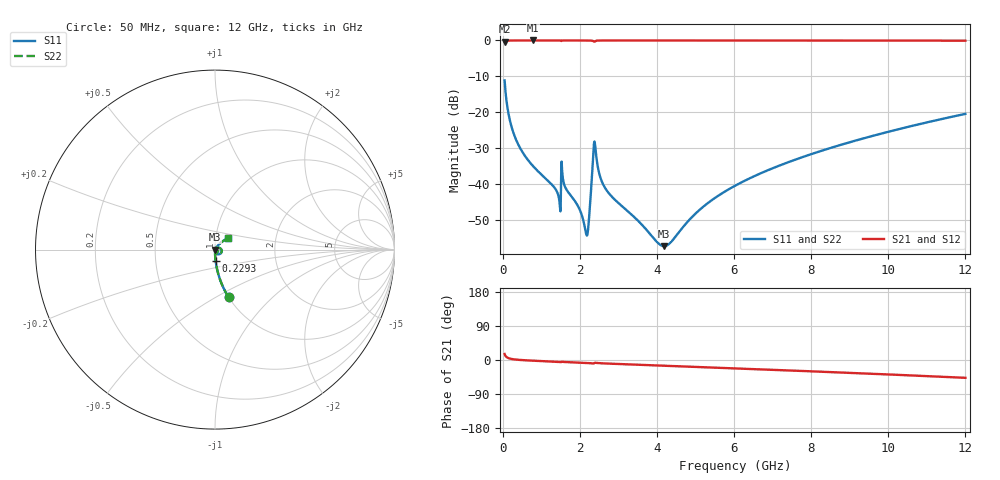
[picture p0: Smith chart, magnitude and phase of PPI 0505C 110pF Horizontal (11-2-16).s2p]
# MHz S MA R 50
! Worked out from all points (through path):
!   1601 points, 50 MHz to 12 GHz, reference 50 ohm
!   highest |S21| = -0.01 dB at 789.4 MHz (marker M1); lowest = -0.3 dB at 50 MHz (marker M2)
!   group delay of S21, straight-line fit = 11.1 ps
!   lowest |S11| = -57.4 dB at 4.188 GHz (marker M3), VSWR 1.00, Z = 50.1 - j0.0392 ohm
!   |S11| at or under -10 dB: start of sweep to end of sweep
!   |S22| runs from -57.4 to -11.1 dB; largest |S21 - S12| = 0
!   S11 on the Smith chart (normalised r, x): 50 MHz: 1.00, -0.58; 229.2 MHz: 1.00, -0.13; 12 GHz: 1.14, +0.14
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50  0.2772 -74.0  0.9606 15.9  0.9606 15.9  0.2772 -74.0
229.25  0.06265 -86.9  0.9976 2.8  0.9976 2.8  0.06265 -86.9
453.3125  0.0315 -88.9  0.9989 0.2  0.9989 0.2  0.0315 -88.9
789.4062  0.01767 -89.7  0.9991 -1.9  0.9991 -1.9  0.01767 -89.7
1319.688  0.0092 -88.8  0.999 -4.3  0.999 -4.3  0.0092 -88.8
1446.656  0.006772 -84.9  0.9987 -4.9  0.9987 -4.9  0.006772 -84.9
1573.625  0.01088 -87.8  0.9985 -5.1  0.9985 -5.1  0.01088 -87.8
2044.156  0.003774 -78.1  0.9986 -7.2  0.9986 -7.2  0.003774 -78.1
2148.719  0.002202 -51.7  0.9983 -7.7  0.9983 -7.7  0.002202 -51.7
2201  0.002021 -4.4  0.9978 -8.0  0.9978 -8.0  0.002021 -4.4
2253.281  0.00418 34.4  0.9968 -8.3  0.9968 -8.3  0.00418 34.4
2342.906  0.02263 27.4  0.9816 -9.3  0.9816 -9.3  0.02263 27.4
2395.188  0.0354 -46.8  0.9723 -7.4  0.9723 -7.4  0.0354 -46.8
2537.094  0.01211 -87.1  0.9974 -8.5  0.9974 -8.5  0.01211 -87.1
2701.406  0.008059 -89.0  0.9983 -9.3  0.9983 -9.3  0.008059 -89.0
4038.312  0.001482 -40.5  0.9984 -14.5  0.9984 -14.5  0.001482 -40.5
4187.688  0.001354 -16.8  0.9984 -15.1  0.9984 -15.1  0.001354 -16.8
5158.625  0.004596 52.2  0.9982 -18.8  0.9982 -18.8  0.004596 52.2
6025  0.009415 57.9  0.9979 -22.1  0.9979 -22.1  0.009415 57.9
8019.156  0.02618 55.7  0.9972 -29.9  0.9972 -29.9  0.02618 55.7
10013.31  0.05348 49.3  0.9956 -38.2  0.9956 -38.2  0.05348 49.3
12000  0.09472 41.3  0.9919 -47.0  0.9919 -47.0  0.09472 41.3
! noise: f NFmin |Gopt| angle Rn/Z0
50  0.0003484  0.8498  0.4011  0.0004941
1372  0.003621  0.6472  5.025  0.001943
2701  0.006372  0.6145  9.834  0.003051
4031  0.007575  0.5409  14.55  0.002885
5360  0.009384  0.5184  19.18  0.003321
6682  0.01117  0.5049  23.67  0.00376
8012  0.01297  0.4974  28.05  0.004215
9341  0.01481  0.4948  32.27  0.004698
1.067e+04  0.01672  0.4962  36.33  0.005225
1.2e+04  0.01874  0.5013  40.22  0.005812
